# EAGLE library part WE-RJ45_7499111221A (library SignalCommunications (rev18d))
Order Code 7499111221A Design THT xBase-T 10/100/1000 Base-T Ports 1x1 Application Standard Tab Position UP LED (Left-Right) GREEN-GREEN EMI Fingers Yes Details see: http://katalog.we-online.de/en/pbs/WE-LAN_RJ45/7499111221A? Updated by Yingchun Shan 2016-08-29 2016(C) Würth Elektronik
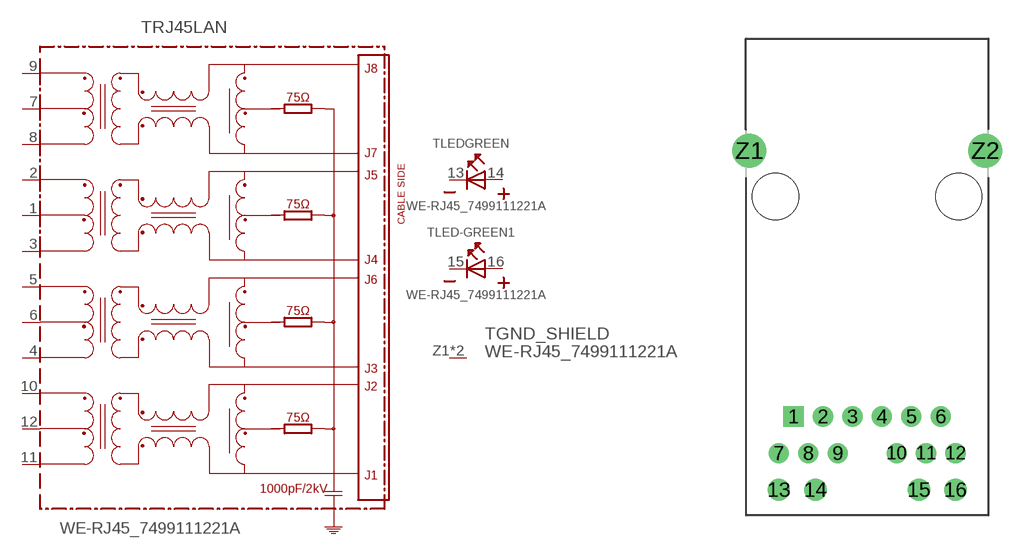
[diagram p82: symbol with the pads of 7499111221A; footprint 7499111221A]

Designator prefix T; gates RJ45LAN=7499111221A/7499111000A LEDGREEN=LED2PIN LED-GREEN1=LED2PIN GND_SHIELD=GNDPIN

## WE-RJ45_7499111221A (COMPANY-URL: http://www.we-online.de; CREATED-BY: Christin Zierenner; CREATED-DATE: AUG 2012; DATASHEET-URL: http://katalog.we-online.de/kataloge/eisos/media/pdf/7499111221A.pdf; MANUFACTURER: Würth Elektronik eiSos GmbH)  [7499111221A]
1  RJ45LAN:1
2  RJ45LAN:2
3  RJ45LAN:3
4  RJ45LAN:4
5  RJ45LAN:5
6  RJ45LAN:6
7  RJ45LAN:7
8  RJ45LAN:8
9  RJ45LAN:9
10  RJ45LAN:10
11  RJ45LAN:11
12  RJ45LAN:12
13  LEDGREEN:K  pas
14  LEDGREEN:A  pas
15  LED-GREEN1:K  pas
16  LED-GREEN1:A  pas
Z1  GND_SHIELD:GND  pwr
Z2  GND_SHIELD:GND  pwr

## Footprint 7499111221A (pad centres in mm)
MAX HEIGHT=15.79mm PORTS----1X1 LED --YES
drill 0.89 square: 1 -5.1,-15.24
drill 0.89: 2 -3.06,-15.24; 3 -1.02,-15.24; 4 1.02,-15.24; 5 3.06,-15.24; 6 5.1,-15.24; 7 -6.12,-17.78; 8 -4.08,-17.78; 9 -2.04,-17.78; 10 2.04,-17.78; 11 4.08,-17.78; 12 6.12,-17.78
drill 1.03: 13 -6.12,-20.32; 14 -3.58,-20.32; 15 3.58,-20.32; 16 6.12,-20.32
drill 1.57: Z1 -8.175,3.18; Z2 8.175,3.18
hole 3.2 at 6.35,0
hole 3.2 at -6.35,0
